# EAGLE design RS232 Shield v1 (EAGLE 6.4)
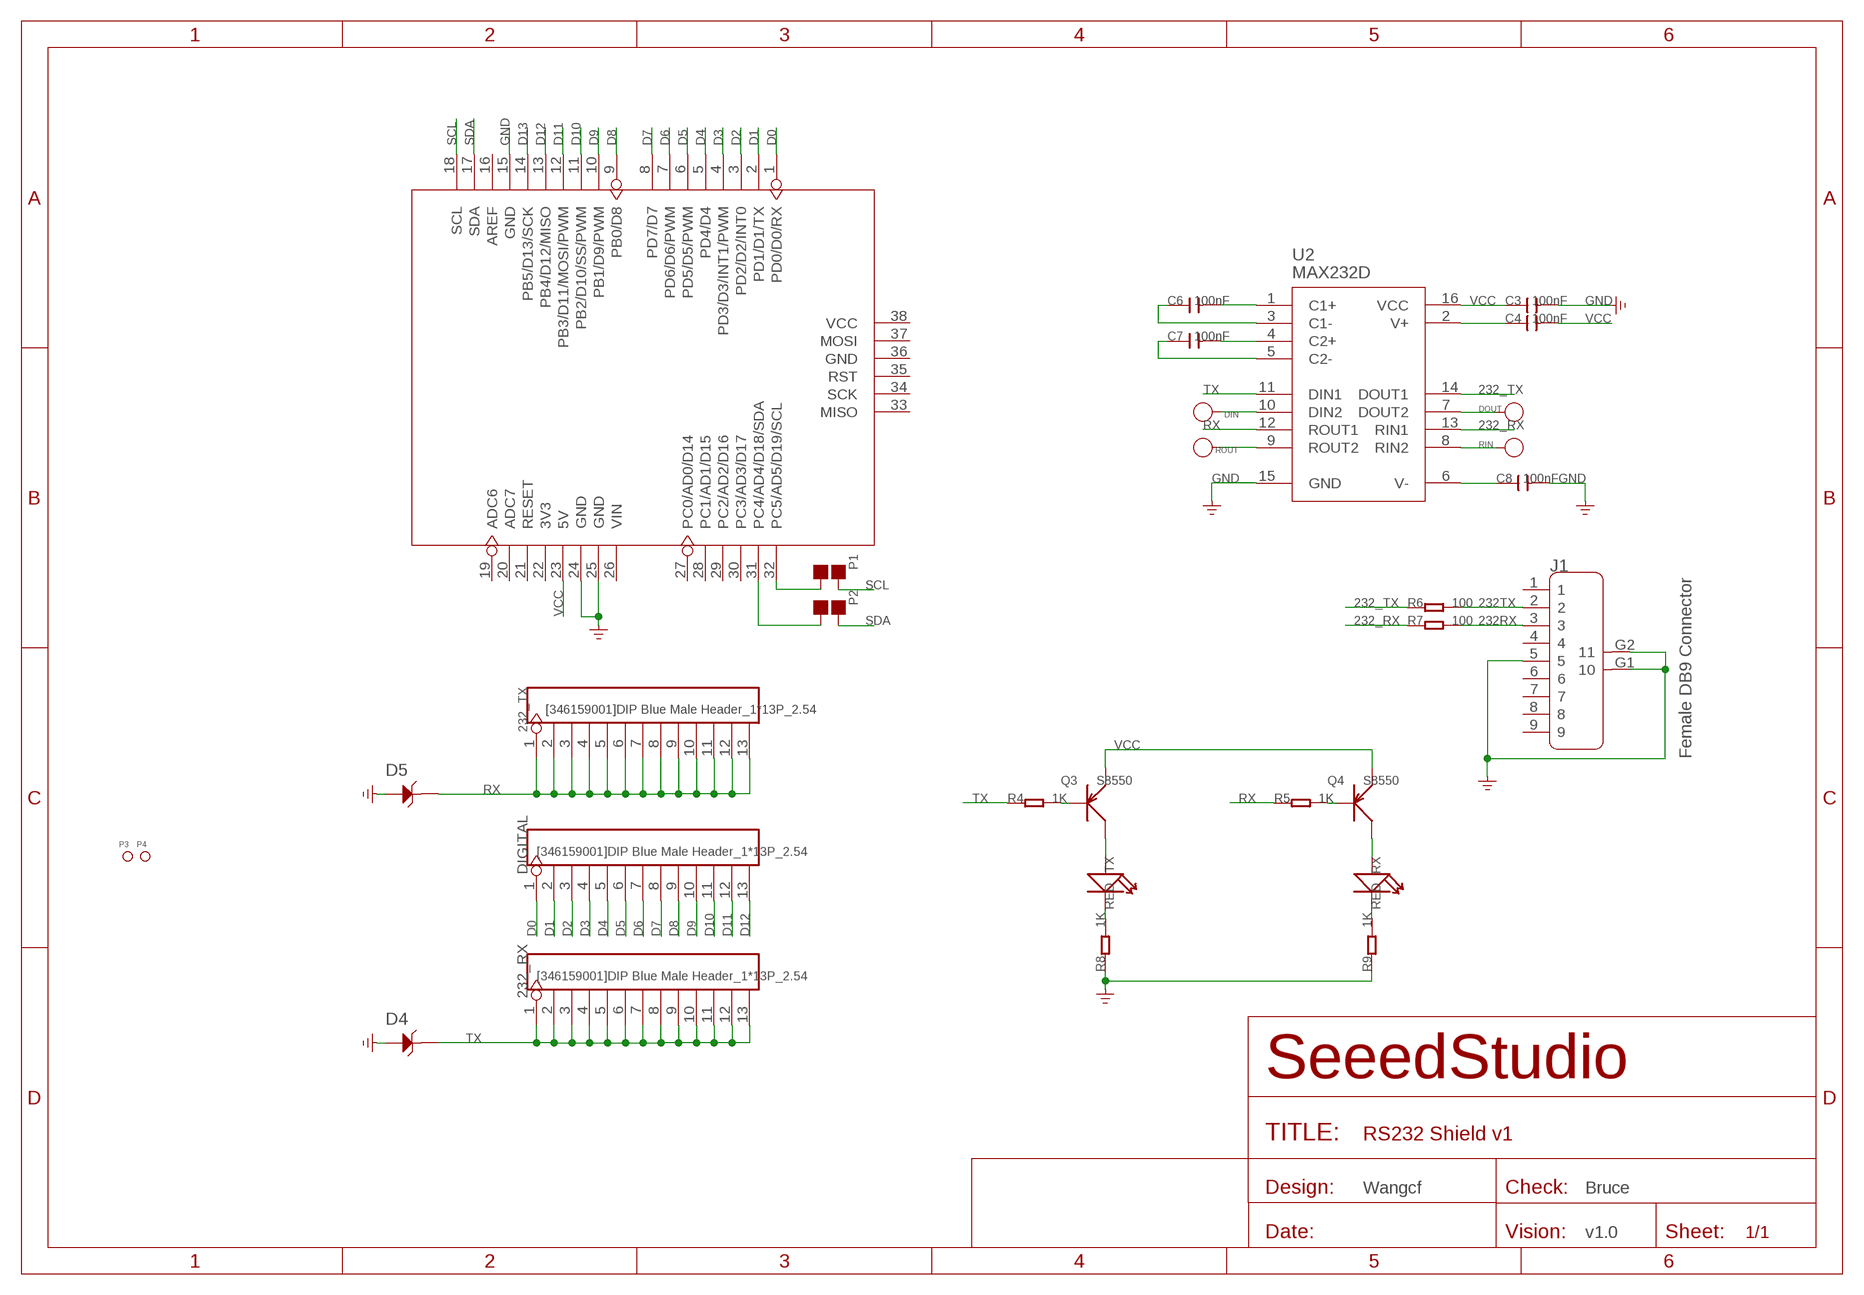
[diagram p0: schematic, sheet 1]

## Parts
232_RX  [346159001]DIP Blue Male Header_1*13P_2.54  HEADER-13P  [13P-2.54]
232_TX  [346159001]DIP Blue Male Header_1*13P_2.54  HEADER-13P  [13P-2.54]
C3  100nF  C-0603  [C0603]
C4  100nF  C-0603  [C0603]
C6  100nF  C-0603  [C0603]
C7  100nF  C-0603  [C0603]
C8  100nF  C-0603  [C0603]
D4  DNP  D-ESD-2P'CESD5V0D1'  [SOD123-2.7X1.6]
D5  DNP  D-ESD-2P'CESD5V0D1'  [SOD123-2.7X1.6]
DIGITAL  [346159001]DIP Blue Male Header_1*13P_2.54  HEADER-13P  [13P-2.54]
DIN  PAD-TEST-POINT'4080'  [PAD_4080]
DOUT  PAD-TEST-POINT'4080'  [PAD_4080]
J1  Female DB9 Connector  DB9'FEMAL'  [DB9]
P1  DNP  PAD-JUMPER-2P  [2P-SMD-1.78X1.27]
P2  DNP  PAD-JUMPER-2P  [2P-SMD-1.78X1.27]
P3  PAD-MARK  [ROUND-MARK-1.0]
P4  PAD-MARK  [ROUND-MARK-1.0]
Q3  S8550  TRANSISTOR-PNP-SOT23  [SOT23]
Q4  S8550  TRANSISTOR-PNP-SOT23  [SOT23]
R4  1K  R-0603  [R0603]
R5  1K  R-0603  [R0603]
R6  100  R-0603  [R0603]
R7  100  R-0603  [R0603]
R8  1K  R-0603  [R0603]
R9  1K  R-0603  [R0603]
RIN  PAD-TEST-POINT'4080'  [PAD_4080]
ROUT  PAD-TEST-POINT'4080'  [PAD_4080]
RX  RED  LED'0603'  [LED-0603]
TX  RED  LED'0603'  [LED-0603]
U1  ARDUINO-38P  [ARDUINO-38P-WITH/-SILK]
U2  MAX232D  MAX3232-SOIC16  [SOIC16]

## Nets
232_RX: R7.1 U2.13(RIN1)
232_TX: R6.1 U2.14(DOUT1)
232RX: J1.3 R7.2
232TX: J1.2 R6.2
D0: DIGITAL.1 U1.1(PD0/D0/RX)
D1: DIGITAL.2 U1.2(PD1/D1/TX)
D2: DIGITAL.3 U1.3(PD2/D2/INT0)
D3: DIGITAL.4 U1.4(PD3/D3/INT1/PWM)
D4: DIGITAL.5 U1.5(PD4/D4)
D5: DIGITAL.6 U1.6(PD5/D5/PWM)
D6: DIGITAL.7 U1.7(PD6/D6/PWM)
D7: DIGITAL.8 U1.8(PD7/D7)
D8: DIGITAL.9 U1.9(PB0/D8)
D9: DIGITAL.10 U1.10(PB1/D9/PWM)
D10: DIGITAL.11 U1.11(PB2/D10/SS/PWM)
D11: DIGITAL.12 U1.12(PB3/D11/MOSI/PWM)
D12: DIGITAL.13 U1.13(PB4/D12/MISO)
D13: U1.14(PB5/D13/SCK)
GND: C3.2 C8.2 D4.1 D5.1 J1.5 J1.G1 J1.G2 R8.1 R9.1 U1.15(GND) U1.24(GND) U1.25(GND) U2.15(GND)
N$1: C6.2 U2.1(C1+)
N$2: P1.1 U1.32(PC5/AD5/D19/SCL)
N$3: C6.1 U2.3(C1-)
N$4: P2.1 U1.31(PC4/AD4/D18/SDA)
N$5: DIN.1(T) U2.10(DIN2)
N$6: ROUT.1(T) U2.9(ROUT2)
N$7: C7.2 U2.4(C2+)
N$8: C7.1 U2.5(C2-)
N$9: C8.1 U2.6(V-)
N$10: C4.1 U2.2(V+)
N$11: Q3.3(C) TX.+
N$14: Q4.3(C) RX.+
N$46: DOUT.1(T) U2.7(DOUT2)
N$47: RIN.1(T) U2.8(RIN2)
N$49: Q3.1(B) R4.2
N$50: Q4.1(B) R5.2
N$51: R8.2 TX.-
N$52: R9.2 RX.-
RX: 232_TX.1 232_TX.2 232_TX.3 232_TX.4 232_TX.5 232_TX.6 232_TX.7 232_TX.8 232_TX.9 232_TX.10 232_TX.11 232_TX.12 232_TX.13 D5.2 R5.1 U2.12(ROUT1)
SCL: P1.2 U1.18(SCL)
SDA: P2.2 U1.17(SDA)
TX: 232_RX.1 232_RX.2 232_RX.3 232_RX.4 232_RX.5 232_RX.6 232_RX.7 232_RX.8 232_RX.9 232_RX.10 232_RX.11 232_RX.12 232_RX.13 D4.2 R4.1 U2.11(DIN1)
VCC: C3.1 C4.2 Q3.2(E) Q4.2(E) U1.23(5V) U2.16(VCC)
Unconnected: J1.1 J1.4 J1.6 J1.7 J1.8 J1.9 U1.16(AREF) U1.19(ADC6) U1.20(ADC7) U1.21(RESET) U1.22(3V3) U1.26(VIN) U1.27(PC0/AD0/D14) U1.28(PC1/AD1/D15) U1.29(PC2/AD2/D16) U1.30(PC3/AD3/D17) U1.33(MISO) U1.34(SCK) U1.35(RST) U1.36(GND) U1.37(MOSI) U1.38(VCC)

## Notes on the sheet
- Wangcf | Bruce
- v1.0

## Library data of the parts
232_RX 232_TX DIGITAL = Connector:HEADER-13P
C3 C4 C6-C8 = Discrete:C*: Ceramic Capacitors
D4 D5 = Discrete:D-ESD-2P: Diodes for Protectiong against ESD
DIN DOUT RIN ROUT = Discrete:PAD-TEST-POINT
J1 = Connector :DB9
P1 P2 = Discrete:PAD-JUMPER-2P; PARTNO: DNP
P3 P4 = Discrete:PAD-MARK; PARTNO: DNP
Q3 Q4 = Discrete:TRANSISTOR-PNP*: PNP audion
R4-R9 = Discrete:R*
RX TX = Discrete:LED*
U1 = moudle:ARDUINO-38P
U2 = IC:MAX3232

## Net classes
0 default: width 0.152 mm, drill 0.305 mm, clearance 0.152 mm

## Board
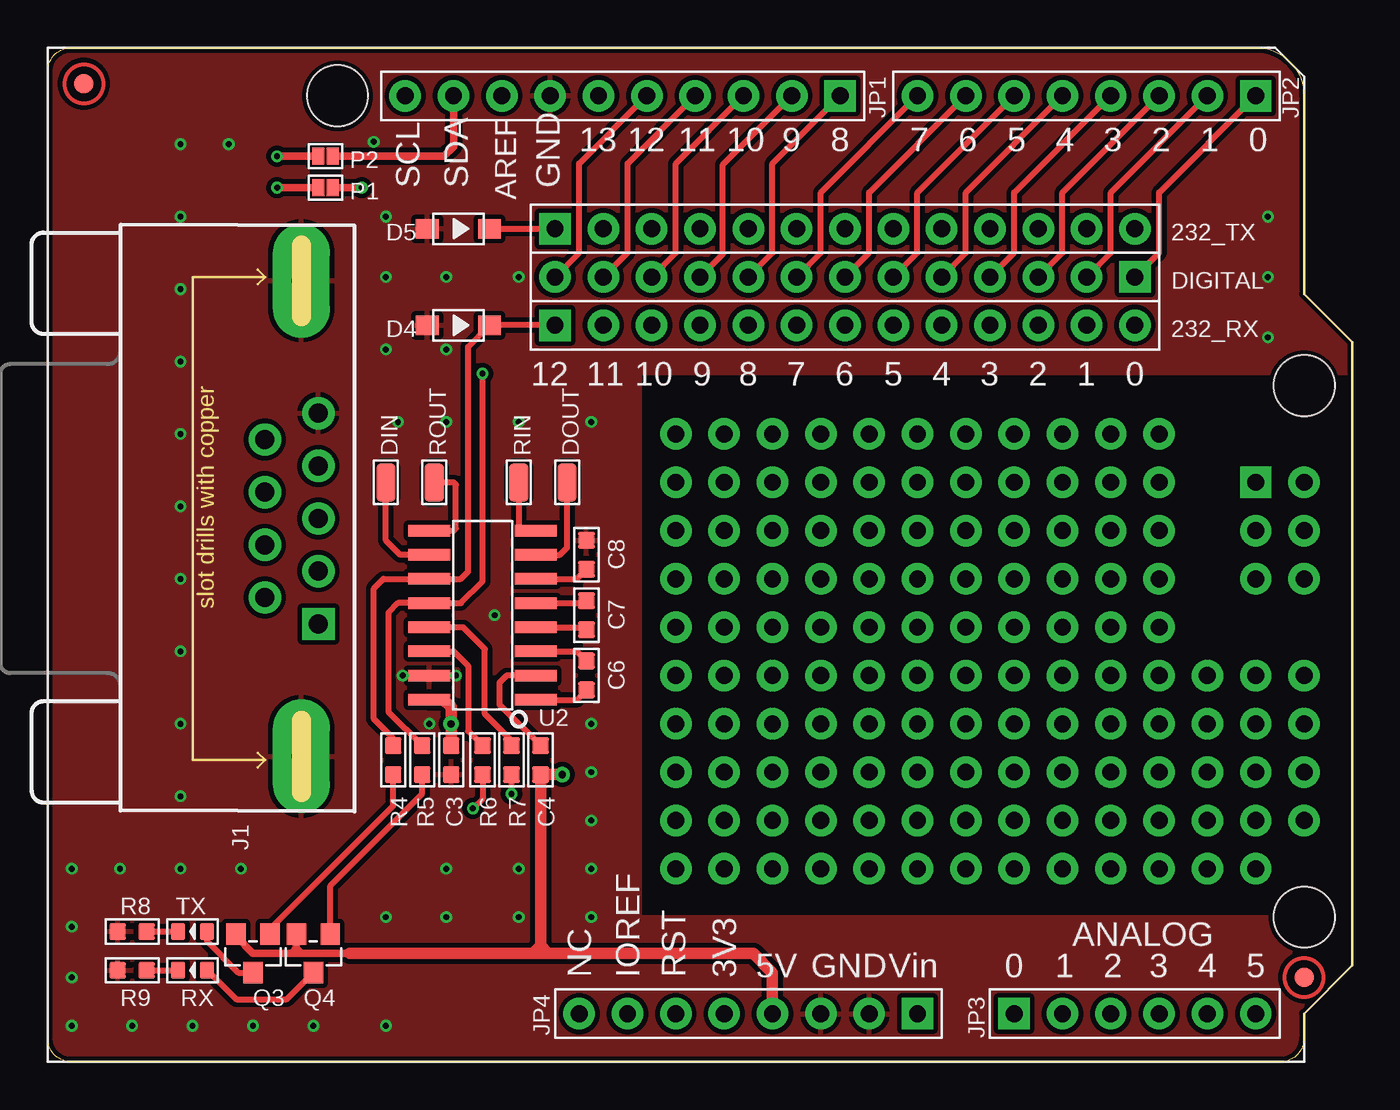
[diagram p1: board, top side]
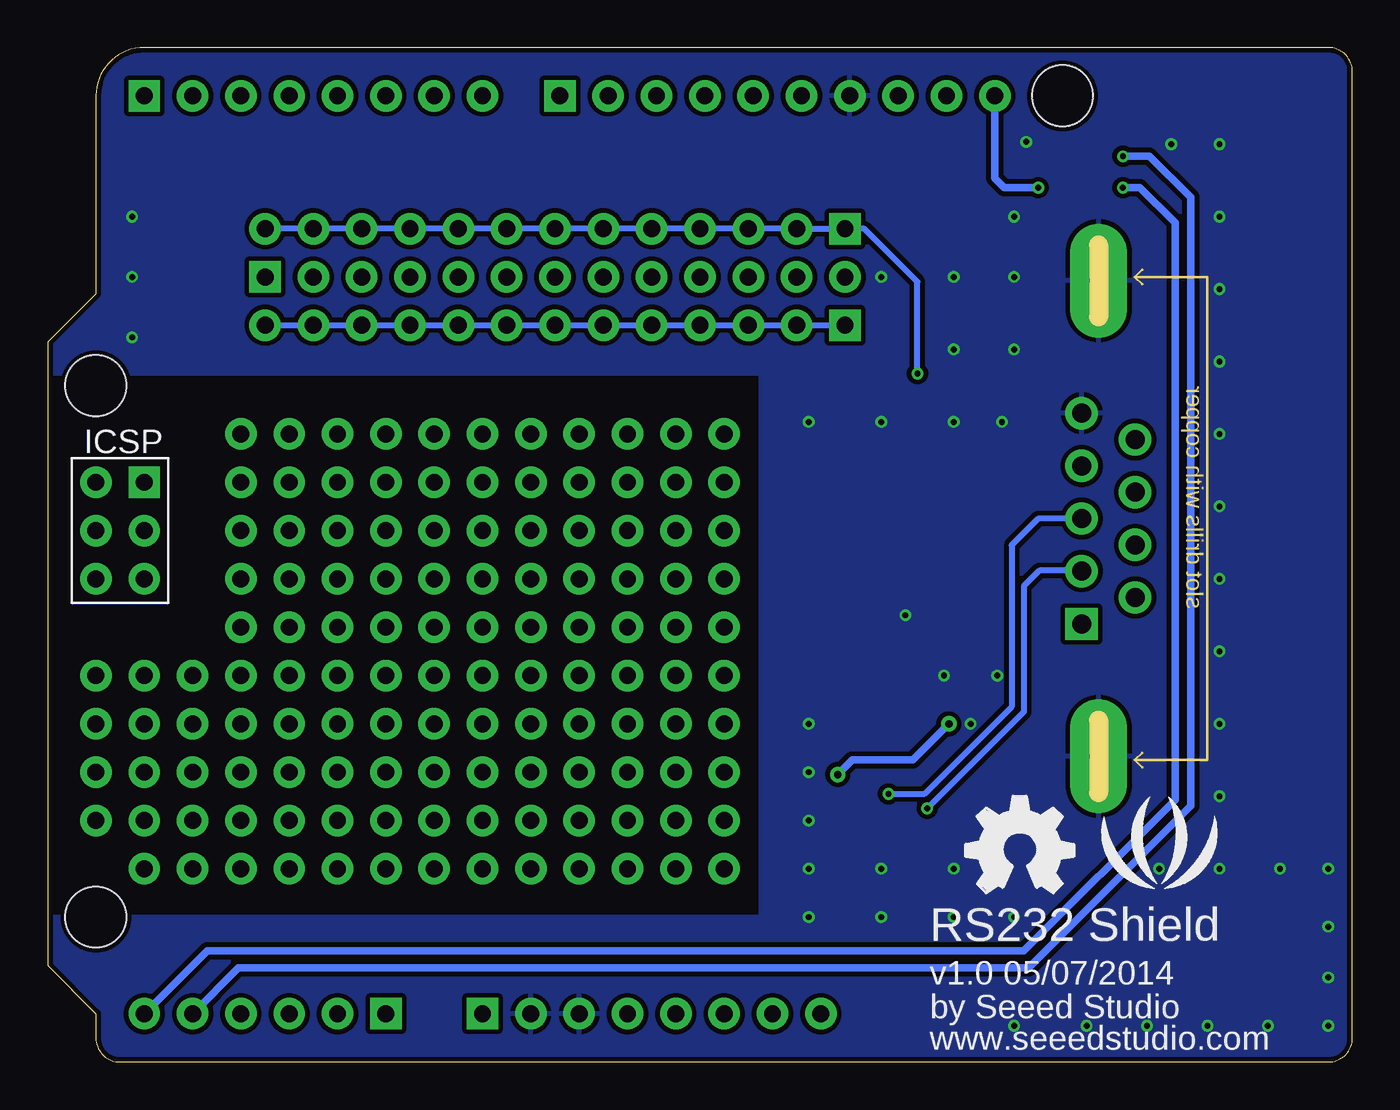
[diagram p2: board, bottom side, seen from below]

Size 68.58 x 53.34 mm. Coordinates in mm from the lower left corner, seen from the top.
Outline: 64.77,0 1.27,0 arc-90 0,1.27 0,52.07 arc-90 1.27,53.34 63.5,53.34 arc-90 66.04,50.8 66.04,40.39 68.58,37.85 68.58,5.08 66.04,2.54 66.04,1.27 arc-90 64.77,0
Copper layers (1*16): Top 0.035mm / dielectric 1.5mm / Bottom 0.035mm
Design rules "SeeedStudio_2layer_DRU_no_angle_20140221 *": minimum track width 6mil, minimum drill 12mil, track to track 6mil, track to pad 6mil, pad to pad 6mil, via to via 6mil, smd to smd 0mil, copper to edge 10mil, drill to drill 10mil, minimum pad ring 10mil, minimum via ring 6mil, stop-mask expansion 2mil, vias tented up to drill 25mil, thermal gap 10mil

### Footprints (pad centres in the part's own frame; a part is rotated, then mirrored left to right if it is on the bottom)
13P-2.54 = drill 0.889 pad 1.651 square: 1 -15.24,0 | drill 0.889 pad 1.651: 2 -12.7,0; 3 -10.16,0; 4 -7.62,0; 5 -5.08,0; 6 -2.54,0; 7 0,0; 8 2.54,0; 9 5.08,0; 10 7.62,0; 11 10.16,0; 12 12.7,0; 13 15.24,0
C0603 = smd 0.889 x 0.889: 1 -0.762,0; 2 0.762,0
SOD123-2.7X1.6 = smd 1.2 x 1.02: 1 -1.635,0; 2 1.635,0
PAD_4080 = smd 2.032 x 1.016: 1 0,0
DB9 = drill 1 pad 1.7 square: 1 5.54,0.9 | drill 1 pad 1.7: 2 2.77,0.9; 3 0,0.9; 4 -2.77,0.9; 5 -5.54,0.9; 6 4.155,-1.91; 7 1.385,-1.91; 8 -1.385,-1.91; 9 -4.155,-1.91 | drill 1 pad 3 long: G1 12.5,0; G2 -12.5,0
2P-SMD-1.78X1.27 = smd 0.889 x 0.61: 1 0,0.381; 2 0,-0.381
ROUND-MARK-1.0 = smd 1.016 x 1.016: P$1 0,0
SOT23 = smd 1.016 x 1.143: 1 -0.889,-1.016; 2 0.889,-1.016; 3 0,1.016
R0603 = smd 0.889 x 0.889: 1 -0.762,0; 2 0.762,0
LED-0603 = smd 0.762 x 0.889: + -0.762,0; - 0.762,0
ARDUINO-38P-WITH/-SILK = drill 0.889 pad 1.651 square: 1 63.5,50.8; 9 41.656,50.8; 26 45.72,2.54; 27 50.8,2.54; 33 63.5,30.48 | drill 0.889 pad 1.651: 2 60.96,50.8; 3 58.42,50.8; 4 55.88,50.8; 5 53.34,50.8; 6 50.8,50.8; 7 48.26,50.8; 8 45.72,50.8; 10 39.116,50.8; 11 36.576,50.8; 12 34.036,50.8; 13 31.496,50.8; 14 28.956,50.8; 15 26.416,50.8; 16 23.876,50.8; 17 21.336,50.8; 18 18.796,50.8; 19 27.94,2.54; 20 30.48,2.54; 21 33.02,2.54; 22 35.56,2.54; 23 38.1,2.54; 24 40.64,2.54; 25 43.18,2.54; 28 53.34,2.54; 29 55.88,2.54; 30 58.42,2.54; 31 60.96,2.54; 32 63.5,2.54; 34 63.5,27.94; 35 63.5,25.4; 36 66.04,25.4; 37 66.04,27.94; 38 66.04,30.48 | hole 3.2: 15.24,50.8; 66.04,35.56; 66.04,7.62
SOIC16 = smd 0.6 x 2.2: 1 -4.445,-2.8; 2 -3.175,-2.8; 3 -1.905,-2.8; 4 -0.635,-2.8; 5 0.635,-2.8; 6 1.905,-2.8; 7 3.175,-2.8; 8 4.445,-2.8; 9 4.445,2.8; 10 3.175,2.8; 11 1.905,2.8; 12 0.635,2.8; 13 -0.635,2.8; 14 -1.905,2.8; 15 -3.175,2.8; 16 -4.445,2.8

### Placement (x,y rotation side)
232_RX  41.91,38.73 0 top
232_TX  41.91,43.81 0 top
C3  21.21,15.88 270 top
C4  25.91,15.88 270 top
C6  28.32,20.32 270 top
C7  28.32,23.5 270 top
C8  28.32,26.67 90 top
D4  21.59,38.73 0 top
D5  21.59,43.81 0 top
DIGITAL  41.91,41.27 180 top
DIN  17.78,30.48 90 top
DOUT  27.3,30.48 90 top
J1  13.34,28.57 270 top
P1  14.61,45.97 90 top
P2  14.61,47.62 90 top
P3  66.04,4.45 0 top
P4  1.91,51.44 0 top
Q3  10.79,5.71 180 top
Q4  13.97,5.71 180 top
R4  18.16,15.88 270 top
R5  19.68,15.88 270 top
R6  22.86,15.88 270 top
R7  24.38,15.88 270 top
R8  4.45,6.86 0 top
R9  4.45,4.83 0 top
RIN  24.77,30.48 90 top
ROUT  20.32,30.48 270 top
RX  7.62,4.83 180 top
TX  7.62,6.86 180 top
U1  0,0 0 top
U2  22.86,23.5 90 top
U$20  [LOGO_SILK]  10.16,10.79 0 bottom
U$47  [OSHW_FILLX200_NOTEXT]  20.32,8.89 0 bottom

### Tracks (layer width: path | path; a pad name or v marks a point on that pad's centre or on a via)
232_RX
  Top 0.305: R7.1 24.38,16.89 22.99,18.29 22.99,21.72 21.84,22.86 U2.13
232_TX
  Top 0.305: U2.14 21.34,21.59 22.1,20.83 22.1,17.4 R6.1
232RX  (via drill 0.3 pad 0.61)
  Top 0.305: v24.38,14.1 R7.2
  Bottom 0.305: J1.3 16.51,28.57 17.91,27.18 17.91,18.67 22.48,14.1 v24.38,14.1
232TX  (via drill 0.3 pad 0.61)
  Top 0.305: R6.2 22.86,13.84 v22.35,13.34
  Bottom 0.305: v22.35,13.34 17.27,18.41 17.27,25.02 16.46,25.83 14.26,25.83 J1.2
D0
  Top 0.305: DIGITAL.1 58.42,42.55 58.42,45.72 U1.1
D1
  Top 0.305: DIGITAL.2 55.88,42.55 55.88,45.72 U1.2
D2
  Top 0.305: DIGITAL.3 53.34,42.55 53.34,45.72 U1.3
D3
  Top 0.305: DIGITAL.4 50.8,42.55 50.8,45.72 U1.4
D4
  Top 0.305: DIGITAL.5 48.26,42.55 48.26,45.72 U1.5
D5
  Top 0.305: DIGITAL.6 45.72,42.55 45.72,45.72 U1.6
D6
  Top 0.305: DIGITAL.7 43.18,42.55 43.18,45.72 U1.7
D7
  Top 0.305: DIGITAL.8 40.64,42.55 40.64,45.72 U1.8
D8
  Top 0.305: DIGITAL.9 38.1,42.55 38.1,47.24 U1.9
D9
  Top 0.305: DIGITAL.10 35.5,42.48 35.5,47.18 U1.10
D10
  Top 0.305: DIGITAL.11 33.02,42.55 33.02,47.24 U1.11
D11
  Top 0.305: DIGITAL.12 30.48,42.55 30.48,47.24 U1.12
D12
  Top 0.305: DIGITAL.13 27.94,42.55 27.94,47.24 U1.13
GND  (via drill 0.3 pad 0.61)
  other vias: 3.81,10.16 17.78,44.45 17.78,41.27 20.95,37.47 20.95,41.27 24.77,41.27 17.78,37.47 18.41,33.66 20.95,33.66 24.77,33.66 28.57,33.66 23.5,23.5 28.57,17.78 28.57,15.24 28.57,12.7 28.57,10.16 28.57,7.62 24.77,7.62 24.77,10.16 20.95,10.16 6.99,10.16 17.78,7.62 10.16,10.16 1.27,10.16 1.27,7.11 1.27,4.45 1.27,1.91 4.45,1.91 7.62,1.91 10.79,1.91 13.97,1.91 17.78,1.91 20.95,7.62 6.99,13.97 6.99,17.78 6.99,21.59 6.99,25.4 6.99,29.21 6.99,33.02 6.99,36.83 6.99,40.64 6.99,44.45 6.99,48.26 9.53,48.26 17.14,48.39 64.14,44.45 64.14,41.27 64.14,38.1 20.07,17.78 18.67,20.32 21.46,20.32
  pour Top (isolate 0.254): 0,53.34 68.58,53.34 68.58,36.2 31.11,36.2 31.11,7.62 68.58,7.62 68.58,0 0,0
  pour Bottom (isolate 0.254): 0,53.34 68.58,53.34 68.58,36.2 31.11,36.2 31.11,7.62 68.58,7.62 68.58,0 0,0
N$1
  Top 0.305: U2.1 27.81,19.05 C6.2
N$2  (via drill 0.3 pad 0.61)
  Top 0.406: P1.1 v12.06,45.97
  Bottom 0.406: U1.32 60.2,5.84 17.26,5.84 9.32,13.78 9.32,44.12 11.18,45.97 v12.06,45.97
N$3
  Top 0.305: U2.3 27.81,21.59 C6.1
N$4  (via drill 0.3 pad 0.61)
  Top 0.406: P2.1 v12.06,47.62
  Bottom 0.406: U1.31 58.55,4.95 17.02,4.95 8.51,13.46 8.51,45.47 10.67,47.62 v12.06,47.62
N$5
  Top 0.305: U2.10 18.54,26.67 17.78,27.43 DIN.1
N$6
  Top 0.305: U2.9 21.34,27.94 21.46,28.07 21.46,30.35 21.34,30.48 ROUT.1
N$7
  Top 0.305: U2.4 28.19,22.86 C7.2
N$8
  Top 0.305: U2.5 28.19,24.13 C7.1
N$9
  Top 0.305: U2.6 27.81,25.4 C8.1
N$10
  Top 0.305: U2.2 24.13,20.32 23.75,19.94 23.75,18.8 C4.1
N$11
  Top 0.305: TX.+ 8.38,6.35 10.03,4.7 Q3.3
N$12  (via drill 0.89 pad 1.65)
  other vias: 33.02,27.94
N$13  (via drill 0.89 pad 1.65)
  other vias: 33.02,25.4
N$14
  Top 0.305: RX.+ 9.91,3.3 12.57,3.3 Q4.3
N$15  (via drill 0.89 pad 1.65)
  other vias: 33.02,22.86
N$16  (via drill 0.89 pad 1.65)
  other vias: 35.56,27.94
N$17  (via drill 0.89 pad 1.65)
  other vias: 35.56,25.4
N$18  (via drill 0.89 pad 1.65)
  other vias: 35.56,22.86
N$19  (via drill 0.89 pad 1.65)
  other vias: 38.1,27.94
N$20  (via drill 0.89 pad 1.65)
  other vias: 38.1,25.4
N$21  (via drill 0.89 pad 1.65)
  other vias: 38.1,22.86
N$22  (via drill 0.89 pad 1.65)
  other vias: 40.64,27.94
N$23  (via drill 0.89 pad 1.65)
  other vias: 40.64,25.4
N$24  (via drill 0.89 pad 1.65)
  other vias: 40.64,22.86
N$25  (via drill 0.89 pad 1.65)
  other vias: 43.18,27.94
N$26  (via drill 0.89 pad 1.65)
  other vias: 43.18,25.4
N$27  (via drill 0.89 pad 1.65)
  other vias: 43.18,22.86
N$28  (via drill 0.89 pad 1.65)
  other vias: 45.72,27.94
N$29  (via drill 0.89 pad 1.65)
  other vias: 45.72,25.4
N$30  (via drill 0.89 pad 1.65)
  other vias: 45.72,22.86
N$31  (via drill 0.89 pad 1.65)
  other vias: 48.26,27.94
N$32  (via drill 0.89 pad 1.65)
  other vias: 48.26,25.4
N$33  (via drill 0.89 pad 1.65)
  other vias: 48.26,22.86
N$34  (via drill 0.89 pad 1.65)
  other vias: 50.8,27.94
N$35  (via drill 0.89 pad 1.65)
  other vias: 50.8,25.4
N$36  (via drill 0.89 pad 1.65)
  other vias: 50.8,22.86
N$37  (via drill 0.89 pad 1.65)
  other vias: 53.34,27.94
N$38  (via drill 0.89 pad 1.65)
  other vias: 53.34,25.4
N$39  (via drill 0.89 pad 1.65)
  other vias: 53.34,22.86
N$40  (via drill 0.89 pad 1.65)
  other vias: 55.88,27.94
N$41  (via drill 0.89 pad 1.65)
  other vias: 55.88,25.4
N$42  (via drill 0.89 pad 1.65)
  other vias: 55.88,22.86
N$43  (via drill 0.89 pad 1.65)
  other vias: 58.42,27.94
N$44  (via drill 0.89 pad 1.65)
  other vias: 58.42,25.4
N$45  (via drill 0.89 pad 1.65)
  other vias: 58.42,22.86
N$46
  Top 0.305: U2.7 26.92,26.67 27.3,27.05 DOUT.1
N$47
  Top 0.305: RIN.1 24.77,28.07 24.89,27.94 U2.8
N$49
  Top 0.305: Q3.1 11.68,6.99 18.16,13.46 R4.2
N$50
  Top 0.305: Q4.1 14.86,9.27 19.68,14.1 R5.2
N$51
  Top 0.305: R8.2 TX.-
N$52
  Top 0.305: R9.2 RX.-
N$54  (via drill 0.89 pad 1.65)
  other vias: 33.02,20.32
N$55  (via drill 0.89 pad 1.65)
  other vias: 33.02,30.48
N$56  (via drill 0.89 pad 1.65)
  other vias: 33.02,17.78
N$57  (via drill 0.89 pad 1.65)
  other vias: 33.02,15.24
N$58  (via drill 0.89 pad 1.65)
  other vias: 35.56,20.32
N$59  (via drill 0.89 pad 1.65)
  other vias: 35.56,17.78
N$60  (via drill 0.89 pad 1.65)
  other vias: 35.56,15.24
N$61  (via drill 0.89 pad 1.65)
  other vias: 38.1,20.32
N$62  (via drill 0.89 pad 1.65)
  other vias: 38.1,17.78
N$63  (via drill 0.89 pad 1.65)
  other vias: 38.1,15.24
N$64  (via drill 0.89 pad 1.65)
  other vias: 40.64,20.32
N$65  (via drill 0.89 pad 1.65)
  other vias: 40.64,17.78
N$66  (via drill 0.89 pad 1.65)
  other vias: 40.64,15.24
N$67  (via drill 0.89 pad 1.65)
  other vias: 43.18,20.32
N$68  (via drill 0.89 pad 1.65)
  other vias: 43.18,17.78
N$69  (via drill 0.89 pad 1.65)
  other vias: 43.18,15.24
N$70  (via drill 0.89 pad 1.65)
  other vias: 45.72,20.32
N$71  (via drill 0.89 pad 1.65)
  other vias: 45.72,17.78
N$72  (via drill 0.89 pad 1.65)
  other vias: 45.72,15.24
N$73  (via drill 0.89 pad 1.65)
  other vias: 48.26,20.32
N$74  (via drill 0.89 pad 1.65)
  other vias: 48.26,17.78
N$75  (via drill 0.89 pad 1.65)
  other vias: 48.26,15.24
N$76  (via drill 0.89 pad 1.65)
  other vias: 50.8,20.32
N$77  (via drill 0.89 pad 1.65)
  other vias: 50.8,17.78
N$78  (via drill 0.89 pad 1.65)
  other vias: 50.8,15.24
N$79  (via drill 0.89 pad 1.65)
  other vias: 53.34,20.32
N$80  (via drill 0.89 pad 1.65)
  other vias: 53.34,17.78
N$81  (via drill 0.89 pad 1.65)
  other vias: 53.34,15.24
N$82  (via drill 0.89 pad 1.65)
  other vias: 55.88,20.32
N$83  (via drill 0.89 pad 1.65)
  other vias: 55.88,17.78
N$84  (via drill 0.89 pad 1.65)
  other vias: 55.88,15.24
N$85  (via drill 0.89 pad 1.65)
  other vias: 58.42,20.32
N$86  (via drill 0.89 pad 1.65)
  other vias: 58.42,17.78
N$87  (via drill 0.89 pad 1.65)
  other vias: 58.42,15.24
N$88  (via drill 0.89 pad 1.65)
  other vias: 60.96,20.32
N$89  (via drill 0.89 pad 1.65)
  other vias: 60.96,17.78
N$90  (via drill 0.89 pad 1.65)
  other vias: 60.96,15.24
N$94  (via drill 0.89 pad 1.65)
  other vias: 33.02,12.7
N$99  (via drill 0.89 pad 1.65)
  other vias: 35.56,30.48
N$100  (via drill 0.89 pad 1.65)
  other vias: 35.56,12.7
N$102  (via drill 0.89 pad 1.65)
  other vias: 63.5,20.32
N$105  (via drill 0.89 pad 1.65)
  other vias: 63.5,17.78
N$106  (via drill 0.89 pad 1.65)
  other vias: 40.64,12.7
N$108  (via drill 0.89 pad 1.65)
  other vias: 63.5,15.24
N$109  (via drill 0.89 pad 1.65)
  other vias: 43.18,12.7
N$111  (via drill 0.89 pad 1.65)
  other vias: 66.04,20.32
N$112  (via drill 0.89 pad 1.65)
  other vias: 45.72,12.7
N$114  (via drill 0.89 pad 1.65)
  other vias: 66.04,17.78
N$115  (via drill 0.89 pad 1.65)
  other vias: 48.26,12.7
N$117  (via drill 0.89 pad 1.65)
  other vias: 66.04,15.24
N$118  (via drill 0.89 pad 1.65)
  other vias: 50.8,12.7
N$120  (via drill 0.89 pad 1.65)
  other vias: 63.5,12.7
N$121  (via drill 0.89 pad 1.65)
  other vias: 53.34,12.7
N$123  (via drill 0.89 pad 1.65)
  other vias: 63.5,10.16
N$124  (via drill 0.89 pad 1.65)
  other vias: 55.88,12.7
N$126  (via drill 0.89 pad 1.65)
  other vias: 66.04,12.7
N$127  (via drill 0.89 pad 1.65)
  other vias: 58.42,12.7
N$130  (via drill 0.89 pad 1.65)
  other vias: 60.96,12.7
N$135  (via drill 0.89 pad 1.65)
  other vias: 35.56,10.16
N$140  (via drill 0.89 pad 1.65)
  other vias: 33.02,10.16
N$143  (via drill 0.89 pad 1.65)
  other vias: 38.1,30.48
N$149  (via drill 0.89 pad 1.65)
  other vias: 60.96,10.16
N$150  (via drill 0.89 pad 1.65)
  other vias: 58.42,10.16
N$151  (via drill 0.89 pad 1.65)
  other vias: 55.88,10.16
N$152  (via drill 0.89 pad 1.65)
  other vias: 53.34,10.16
N$153  (via drill 0.89 pad 1.65)
  other vias: 50.8,10.16
N$154  (via drill 0.89 pad 1.65)
  other vias: 48.26,10.16
N$155  (via drill 0.89 pad 1.65)
  other vias: 43.18,10.16
N$156  (via drill 0.89 pad 1.65)
  other vias: 33.02,33.02
N$157  (via drill 0.89 pad 1.65)
  other vias: 35.56,33.02
N$158  (via drill 0.89 pad 1.65)
  other vias: 38.1,33.02
N$159  (via drill 0.89 pad 1.65)
  other vias: 40.64,33.02
N$160  (via drill 0.89 pad 1.65)
  other vias: 43.18,33.02
N$161  (via drill 0.89 pad 1.65)
  other vias: 45.72,33.02
N$162  (via drill 0.89 pad 1.65)
  other vias: 48.26,33.02
N$163  (via drill 0.89 pad 1.65)
  other vias: 50.8,33.02
N$164  (via drill 0.89 pad 1.65)
  other vias: 53.34,33.02
N$165  (via drill 0.89 pad 1.65)
  other vias: 55.88,33.02
N$166  (via drill 0.89 pad 1.65)
  other vias: 58.42,33.02
N$182  (via drill 0.89 pad 1.65)
  other vias: 38.1,12.7
N$183  (via drill 0.89 pad 1.65)
  other vias: 38.1,10.16
N$184  (via drill 0.89 pad 1.65)
  other vias: 40.64,10.16
N$187  (via drill 0.89 pad 1.65)
  other vias: 40.64,30.48
N$231  (via drill 0.89 pad 1.65)
  other vias: 43.18,30.48
N$275  (via drill 0.89 pad 1.65)
  other vias: 45.72,30.48
N$319  (via drill 0.89 pad 1.65)
  other vias: 48.26,30.48
N$363  (via drill 0.89 pad 1.65)
  other vias: 50.8,30.48
N$407  (via drill 0.89 pad 1.65)
  other vias: 53.34,30.48
N$451  (via drill 0.89 pad 1.65)
  other vias: 55.88,30.48
N$495  (via drill 0.89 pad 1.65)
  other vias: 58.42,30.48
N$539  (via drill 0.89 pad 1.65)
  other vias: 45.72,10.16
RX  (via drill 0.3 pad 0.61)
  Top 0.305: 232_TX.1 D5.2 23.5,43.81 | R5.1 17.91,18.41 17.91,23.62 18.41,24.13 U2.12 21.72,24.13 22.86,25.27 v22.86,36.2
  Bottom 0.305: 232_TX.13 232_TX.12 232_TX.11 232_TX.10 232_TX.9 232_TX.8 232_TX.7 232_TX.6 232_TX.5 232_TX.4 232_TX.3 232_TX.2 232_TX.1 25.65,43.81 22.86,41.02 v22.86,36.2
SCL  (via drill 0.3 pad 0.61)
  Top 0.406: P1.2 v16.51,45.97
  Bottom 0.406: U1.18 18.8,46.48 18.29,45.97 v16.51,45.97
SDA
  Top 0.406: P2.2 20.83,47.62 21.34,48.13 U1.17
TX
  Top 0.305: 232_RX.1 D4.2 22.1,37.61 22.1,25.78 21.72,25.4 U2.11 17.65,25.4 17.14,24.89 17.14,18.03 18.16,17.02 R4.1
  Bottom 0.305: 232_RX.13 232_RX.12 232_RX.11 232_RX.10 232_RX.9 232_RX.8 232_RX.7 232_RX.6 232_RX.5 232_RX.4 232_RX.3 232_RX.2 232_RX.1
VCC  (via drill 0.38 pad 0.81)
  Top 0.406: Q3.2 9.91,6.6 10.79,5.71 12.83,5.71 | 12.83,5.71 13.34,5.71 | 13.34,5.71 15.88,5.71 | Q4.2 13.08,5.97 | 13.08,5.97 12.83,5.71 | 13.08,5.97 13.34,5.71
  Top 0.61: U2.16 20.83,19.05 21.21,18.67 v21.21,17.78 C3.1 | U1.23 38.1,4.7 37.08,5.71 26.29,5.71 | v27.05,15.11 C4.2 25.91,6.1 | 15.88,5.71 25.53,5.71 | 25.53,5.71 26.29,5.71 | 25.91,6.1 25.53,5.71 | 25.91,6.1 26.29,5.71
  Bottom 0.406: v21.21,17.78 23.11,15.88 26.29,15.88 v27.05,15.11

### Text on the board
tPlace: JP1 | JP2 | 12 | 11 | 10 | 9 | 8 | 7 | 6 | 5 | 4 | 3 | 2 | 1 | 0 | JP4 | JP3
bPlace: ICSP | RS232 Shield | v1.0 05/07/2014 | by Seeed Studio | www.seeedstudio.com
